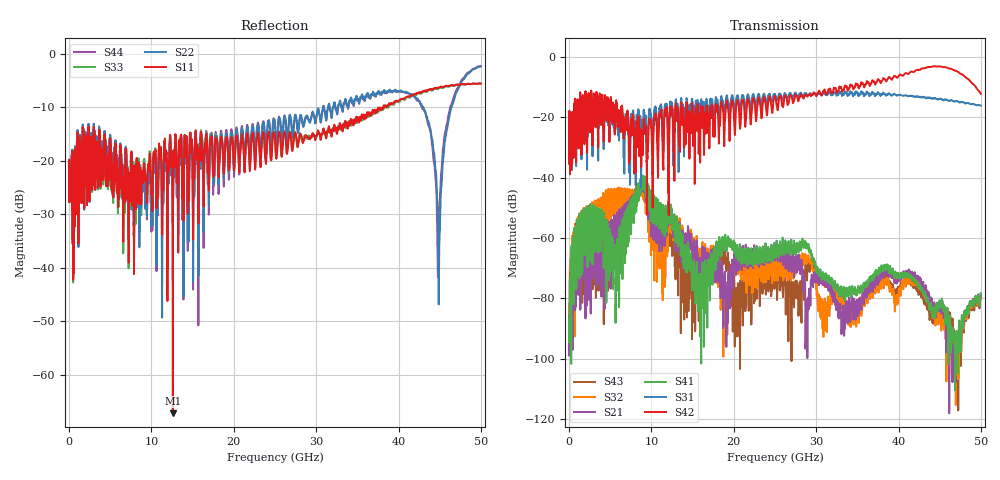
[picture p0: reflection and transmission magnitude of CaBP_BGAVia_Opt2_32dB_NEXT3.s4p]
!* Samtec Inc. NovaRay Examax Flyover System  *
!*  REV DATE  = 08/08/18  *
!*  TYPE  = TOUCHSTONE  *
!*  PORTS  = 4 port  *
!*  UNITS  = GHz  *
!*  DATA RANGE = DC  to 50 GHz; 10 MHz Step  *
!*  PARAMETER  = S  *
!*  FORMAT  = Real-Imaginary  *
!*  REFERENCE  = 50 ohms  *
!*  SOURCE  = HFSS  *
!*  VALIDATED  = No  *
!*  MANUFACTURER = SAMTEC  *
!*  INTERCONNECT = NVAx to EBCx to EBCx to NVAx  *
!*  [Full Channel NVAx to EBCx to EBCx to NVAx  with PCB Trace and BGA Via]  *
!*  BOUNDARY A  = Silicon BGA Ball Pad  *
!*  BOUNDARY B  = Silicon BGA Ball Pad  *
!*  NVAx (end a) ->>- (end b) NVAx  *
!*  Port 01 ->>- Port 02  *
!*  Port 03 ->>- Port 04  *
!***************************** CHANNEL MODEL ******************************************
# GHz S RI R 50
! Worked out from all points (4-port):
!   5000 points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, 10 MHz to 50 GHz, reference 50 ohm
!   strongest paths, dB at 10 MHz, 12.51 GHz, 25.01 GHz, 37.51 GHz, 50 GHz:
!     S42: -23.1, -16.4, -12.8, -7.3, -12.2
!     S31: -23.1, -15.2, -12.2, -11.7, -16.1
!     S41: -90.2, -54.8, -64.3, -71.3, -78.5
!     S21: -99.0, -54.3, -65.3, -74.5, -78.9
!     S32: -90.6, -54.4, -70.2, -76.7, -79.6
!     S43: -96.0, -64.9, -72.9, -73.5, -79.4
!   lowest |S11| = -67.2 dB at 12.6 GHz (marker M1), VSWR 1.00, Z = 50 + j0.0147 ohm
!   |S11| at or under -10 dB: start of sweep to 37.74 GHz; 37.74 GHz to 38.13 GHz (385.5 MHz wide, 1.02 % of centre); 38.51568 GHz to 38.54961 GHz (33.93 MHz wide, 0.0881 % of centre)
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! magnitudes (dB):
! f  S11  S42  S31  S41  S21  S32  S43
! 10 MHz  -21.6  -23.1  -23.1  -90.2  -99.0  -90.6  -96.0
! 8.83 GHz  -23.3  -25.7  -22.2  -39.7  -41.2  -44.4  -40.4
! 12.6 GHz  -67.2  -20.3  -21.8  -55.3  -55.8  -55.7  -65.2
! 15.89 GHz  -20.0  -25.1  -19.2  -72.1  -66.6  -63.5  -68.8
! 40.3 GHz  -8.5  -5.9  -12.6  -71.9  -72.5  -76.8  -75.2
! 44.9 GHz  -6.3  -3.1  -13.8  -81.3  -83.7  -86.3  -82.7
! 50 GHz  -5.5  -12.2  -16.1  -78.5  -78.9  -79.6  -79.4
